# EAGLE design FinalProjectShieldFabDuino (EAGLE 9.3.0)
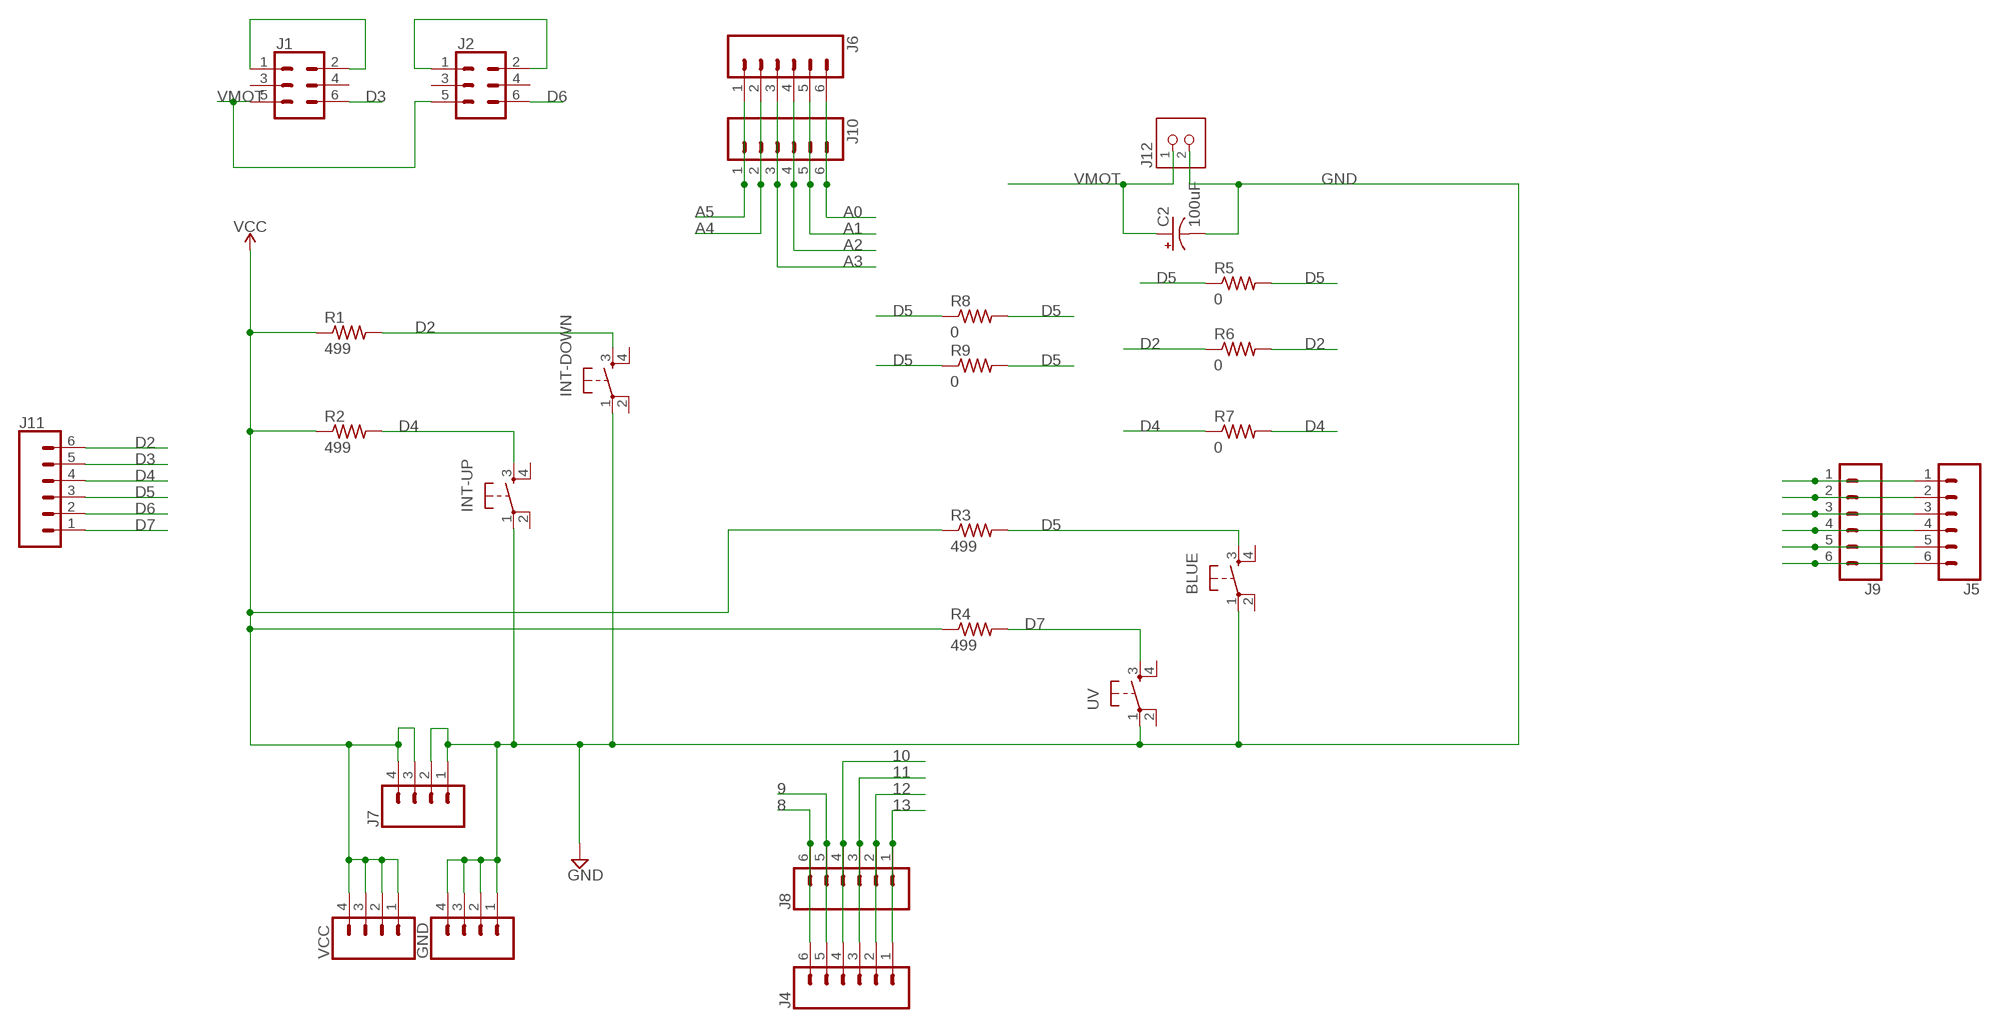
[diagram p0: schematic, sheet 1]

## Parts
BLUE  6MM_SWITCH6MM_SWITCH  [6MM_SWITCH]
C2  100uF  SPARKFUN-CAPACITORS_100UF-POLAR-RADIAL-2.5MM-25V-20%  [SPARKFUN-CAPACITORS_CPOL-RADIAL-2.5MM-6.5MM]
GND  CONN_04PTH  [1X04]
INT-DOWN  6MM_SWITCH6MM_SWITCH  [6MM_SWITCH]
INT-UP  6MM_SWITCH6MM_SWITCH  [6MM_SWITCH]
J1  CONN_03X2FEMALE_SMD  [2X3_SMD]
J2  CONN_03X2FEMALE_SMD  [2X3_SMD]
J4  CONN_06SILK_FEMALE_PTH  [1X06]
J5  CONN_06SILK_FEMALE_PTH  [1X06]
J6  CONN_06SILK_FEMALE_PTH  [1X06]
J7  SPARKFUN-CONNECTORS_CONN_04PTH  [SPARKFUN-CONNECTORS_1X04]
J8  CONN_06FEMALE_LOCK  [1X06_FEMALE_LOCK.010]
J9  CONN_06FEMALE_LOCK  [1X06_FEMALE_LOCK.010]
J10  CONN_06FEMALE_LOCK  [1X06_FEMALE_LOCK.010]
J11  CONN_06FEMALE_LOCK  [1X06_FEMALE_LOCK.010]
J12  FAB_TERM-1X02-ADAFRUIT  [FAB_3.5MMTERM]
R1  499  RES-US1206FAB  [R1206FAB]
R2  499  RES-US1206FAB  [R1206FAB]
R3  499  RES-US1206FAB  [R1206FAB]
R4  499  RES-US1206FAB  [R1206FAB]
R5  0  RES-US1206FAB  [R1206FAB]
R6  0  RES-US1206FAB  [R1206FAB]
R7  0  RES-US1206FAB  [R1206FAB]
R8  0  RES-US1206FAB  [R1206FAB]
R9  0  RES-US1206FAB  [R1206FAB]
UV  6MM_SWITCH6MM_SWITCH  [6MM_SWITCH]
VCC  CONN_04PTH  [1X04]

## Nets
8: J4.6 J8.6
9: J4.5 J8.5
10: J4.4 J8.4
11: J4.3 J8.3
12: J4.2 J8.2
13: J4.1 J8.1
A0: J6.6 J10.6
A1: J6.5 J10.5
A2: J6.4 J10.4
A3: J6.3 J10.3
A4: J6.2 J10.2
A5: J6.1 J10.1
D2: INT-DOWN.3(S) J11.6 R1.2 R6.1 R6.2
D3: J1.6 J11.5
D4: INT-UP.3(S) J11.4 R2.2 R7.1 R7.2
D5: BLUE.3(S) J11.3 R3.2 R5.1 R5.2 R8.1 R8.2 R9.1 R9.2
D6: J2.6 J11.2
D7: J11.1 R4.2 UV.3(S)
GND: BLUE.1(P) C2.2(-) GND.1 GND.2 GND.3 GND.4 INT-DOWN.1(P) INT-UP.1(P) J7.1 J7.2 J12.2 UV.1(P)
N$1: J1.1 J1.2
N$2: J2.1 J2.2
N$13: J5.1 J9.1
N$14: J5.2 J9.2
N$15: J5.3 J9.3
N$16: J5.4 J9.4
N$17: J5.5 J9.5
N$18: J5.6 J9.6
VCC: J7.3 J7.4 R1.1 R2.1 R3.1 R4.1 VCC.1 VCC.2 VCC.3 VCC.4
VMOT: C2.1(+) J1.5 J2.5 J12.1
Unconnected: BLUE.2(P1) BLUE.4(S1) INT-DOWN.2(P1) INT-DOWN.4(S1) INT-UP.2(P1) INT-UP.4(S1) J1.3 J1.4 J2.3 J2.4 UV.2(P1) UV.4(S1)

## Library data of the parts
BLUE INT-DOWN INT-UP UV = fab:6MM_SWITCH: OMRON SWITCH
C2 = GRBLShieldFabDuino:SPARKFUN-CAPACITORS_100UF-POLAR: 100µF polarized capacitors; PROD_ID: CAP-08439
GND VCC = SparkFun-Connectors:CONN_04: Multi connection point. Often used as Generic Header-pin footprint for 0.1 inch spaced/style header connections On any of the 0.1 inch spaced packages, you can populate with these: Break Away Headers - Straight (PRT-00116) Break Away Male Headers - Right Angle (PRT-00553) Female Headers (PRT-00115)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; PROD_ID: CONN-09696
J1 J2 = fab:CONN_03X2: Multi connection point. Often used as Generic Header-pin footprint for 0.1 inch spaced/style header connections You can populate with any combo of single row headers, but if you'd like an exact match, check these: Header - 2x3 (Male, 0.1") (PRT-12807) Header - 2x3 (Female, 0.1") (PRT-13010) 2x3 Pin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; PROD_ID: CONN-11290
J4-J6 = SparkFun-Connectors:CONN_06: Multi connection point. Often used as Generic Header-pin footprint for 0.1 inch spaced/style header connections On any of the 0.1 inch spaced packages, you can populate with these: Break Away Headers - Straight (PRT-00116) Break Away Male Headers - Right Angle (PRT-00553) Female Headers (PRT-00115)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; PROD_ID: CONN-08437
J7 = GRBLShieldFabDuino:SPARKFUN-CONNECTORS_CONN_04: Multi connection point. Often used as Generic Header-pin footprint for 0.1 inch spaced/style header connections On any of the 0.1 inch spaced packages, you can populate with these: Break Away Headers - Straight (PRT-00116) Break Away Male Headers - Right Angle (PRT-00553) Female Headers (PRT-00115)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; PROD_ID: CONN-09696
J8-J11 = SparkFun-Connectors:CONN_06: Multi connection point. Often used as Generic Header-pin footprint for 0.1 inch spaced/style header connections On any of the 0.1 inch spaced packages, you can populate with these: Break Away Headers - Straight (PRT-00116) Break Away Male Headers - Right Angle (PRT-00553) Female Headers (PRT-00115)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
J12 = GRBLShieldFabDuino:FAB_TERM-1X02: 3.5mm terminal block, 2 positions ED555-2DS as found in the fablab inventory.
R1-R9 = fab:RES-US: Resistor (US Symbol)

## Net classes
0 default: clearance 0.406 mm

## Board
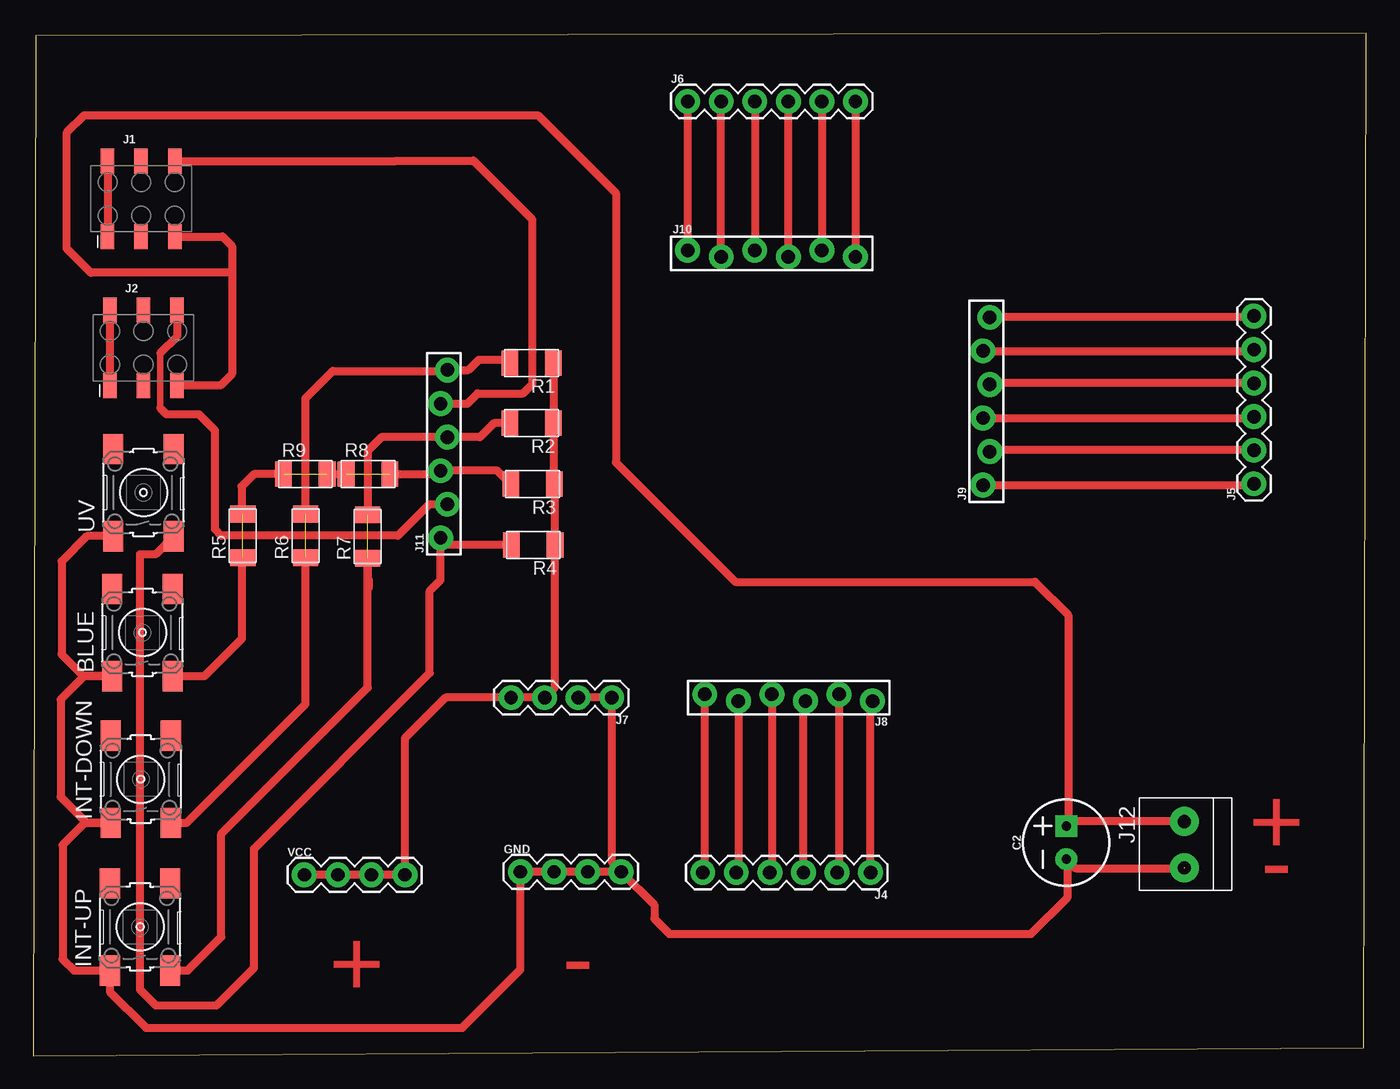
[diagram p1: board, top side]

Size 100.89 x 77.39 mm. Coordinates in mm from the lower left corner, seen from the top.
Outline: 0,0 100.69,0.61 100.89,77.39 0.2,77.19 0,0
Copper layers (1*16): Top 0.035mm / dielectric 1.5mm / Bottom 0.035mm
Design rules "default": minimum track width 6mil, minimum drill 0.35mm, track to track 6mil, track to pad 6mil, pad to pad 6mil, via to via 6mil, smd to smd 6mil, copper to edge 40mil, drill to drill 6mil, minimum pad ring 10mil, minimum via ring 8mil, stop-mask expansion 4mil, vias tented up to drill 0mil, thermal gap 10mil

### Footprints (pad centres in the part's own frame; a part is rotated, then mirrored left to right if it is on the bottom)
6MM_SWITCH = smd 2.286 x 1.524: 1 -3.302,2.286; 2 3.302,2.286; 3 -3.302,-2.286; 4 3.302,-2.286
SPARKFUN-CAPACITORS_CPOL-RADIAL-2.5MM-6.5MM = drill 0.7 pad 1.651 square: 1 1.25,0 | drill 0.7 pad 1.651: 2 -1.25,0
1X04 = drill 1.016 pad 1.88: 1 0,0; 2 2.54,0; 3 5.08,0; 4 7.62,0
2X3_SMD = smd 1.02 x 1.9: 1 -2.54,-2.85; 2 -2.54,2.85; 3 0,-2.85; 4 0,2.85; 5 2.54,-2.85; 6 2.54,2.85
1X06 = drill 1.016 pad 1.88: 1 0,0; 2 2.54,0; 3 5.08,0; 4 7.62,0; 5 10.16,0; 6 12.7,0
SPARKFUN-CONNECTORS_1X04 = drill 1.016 pad 1.88: 1 0,0; 2 2.54,0; 3 5.08,0; 4 7.62,0
1X06_FEMALE_LOCK.010 = drill 1.016 pad 1.88: 1 0,0.254; 2 2.54,-0.254; 3 5.08,0.254; 4 7.62,-0.254; 5 10.16,0.254; 6 12.7,-0.254
FAB_3.5MMTERM = drill 1 pad 2.184: 1 1.8,0; 2 -1.7,0
R1206FAB = smd 1.27 x 1.905: 1 -1.651,0; 2 1.651,0

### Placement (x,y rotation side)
BLUE  8.28,32.03 90 top
C2  78.18,16.13 90 top
GND  36.88,13.92 0 top
INT-DOWN  8.15,20.93 90 top
INT-UP  8.1,9.75 90 top
J1  8.18,64.85 0 top
J2  8.36,53.57 0 top
J4  63.37,13.87 180 top
J5  92.38,43.28 90 top
J6  49.53,72.21 0 top
J7  43.79,27.1 180 top
J8  63.53,27.1 180 top
J9  72.14,43.18 90 top
J10  49.53,60.71 0 top
J11  31.09,39.19 90 top
J12  87.12,15.93 90 top
R1  37.72,52.43 180 top
R2  37.72,47.88 180 top
R3  37.8,43.26 180 top
R4  37.85,38.66 180 top
R5  15.88,39.34 90 top
R6  20.62,39.34 90 top
R7  25.32,39.29 90 top
R8  25.35,44.02 0 top
R9  20.6,44.02 0 top
UV  8.36,42.62 90 top
VCC  20.52,13.69 0 top

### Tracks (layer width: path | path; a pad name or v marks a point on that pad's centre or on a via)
8
  Top 0.61: J4.6 50.83,14.02 J8.6
9
  Top 0.61: J8.5 53.37,14.02 J4.5
10
  Top 0.61: J8.4 55.91,14.02 J4.4
11
  Top 0.61: J4.3 58.29,26.7 J8.3
12
  Top 0.61: J8.2 60.99,14.27 61.39,13.87 61.39,13.97 61.29,13.87 J4.2
13
  Top 0.61: J4.1 63.37,26.7 J8.1
A0
  Top 0.61: J6.6 J10.6
A1
  Top 0.61: J6.5 J10.5
A2
  Top 0.61: J10.4 J6.4
A3
  Top 0.61: J6.3 J10.3
A4
  Top 0.61: J10.2 J6.2
A5
  Top 0.61: J6.1 J10.1
D2  (1 unrouted)
  Top 0.61: R1.2 35.81,52.68 33.73,52.68 32.94,51.89 J11.6 31.27,51.82 22.68,51.82 20.62,49.76 R6.2 | INT-DOWN.3 11.63,17.63 20.62,26.62 R6.1
D3
  Top 0.61: J1.6 26.59,67.7 27.38,67.7 33.28,67.7 33.32,67.74 37.79,63.27 37.79,50.83 37.08,50.11 33.63,50.11 32.87,49.35 J11.5
D4  (1 unrouted)
  Top 0.61: R2.2 34.87,47.88 33.81,46.81 J11.4 26.36,46.81 25.32,45.77 R7.2 | INT-UP.3 11.71,6.45 14.25,8.99 14.25,16.8 25.32,27.87 R7.1 25.32,35.51 25.43,35.41 25.43,36.02
D5  (3 unrouted)
  Top 0.61: R3.2 35.13,44.27 J11.3 30.58,44.02 R8.2 | BLUE.3 12.98,28.73 15.8,31.55 15.8,37.62 R5.1 | R9.1 16.71,44.02 15.77,43.08 15.77,41.1 R5.2 | R9.2 R8.1
D6
  Top 0.508: 9.62,53.16 9.62,49.02
  Top 0.61: J2.6 10.9,54.43 9.62,53.16 | 9.62,49.02 10.09,48.55 12.54,48.55 13.77,47.32 13.77,39.85 14.25,39.37 27.61,39.37 29.97,41.73 J11.2 31.32,41.71
D7
  Top 0.61: R4.2 31.37,38.66 J11.1 | 10.87,39.24 10.79,39.32 UV.3 9.27,37.95 8.08,37.95 8.08,5.03 9.3,3.81 13.89,3.81 16.73,6.64 16.73,15.66 30.02,28.96 30.02,35.18 30.84,35.99 J11.1 | 30.78,39.24 J11.1
GND  (1 unrouted)
  Top 0.61: C2.2 78.29,14.77 | 78.29,14.77 78.86,14.2 87.15,14.2 87.2,14.15 | GND.4 GND.3 GND.2 GND.1 36.88,6.53 32.47,2.12 8.55,2.12 5.82,4.85 INT-UP.1 3.1,6.45 2.23,7.31 2.23,15.95 3.91,17.63 INT-DOWN.1 4.06,17.63 2.08,19.61 2.08,26.95 3.86,28.73 BLUE.1 3.81,28.73 2.16,30.38 2.16,37.41 4.06,39.32 UV.1 | GND.4 44.5,13.97 43.79,14.68 J7.1 J7.2 | GND.4 47.02,11.4 47.02,10.36 48.16,9.22 75.51,9.22 78.29,12 78.29,14.77
N$1
  Top 0.61: J1.2 J1.1
N$2
  Top 0.61: J2.2 J2.1
N$13
  Top 0.61: J9.1 92.28,43.18 J5.1
N$14
  Top 0.61: J5.2 72.49,45.82 J9.2
N$15
  Top 0.61: J9.3 92.28,48.26 J5.3
N$16
  Top 0.61: J5.4 72.49,50.9 J9.4
N$17
  Top 0.61: J9.5 92.91,53.34 92.94,53.37 92.86,53.44 J5.5
N$18
  Top 0.61: J5.6 92.28,55.88 J9.6
VCC
  Top 0.61: VCC.1 VCC.2 VCC.3 VCC.4 28.12,13.72 28.12,24 31.22,27.1 J7.4 J7.3 39.5,27.89 R4.1 39.45,38.71 R3.1 39.37,43.33 R2.1 R1.1
VMOT
  Top 0.61: 78.33,17.53 78.53,17.73 J12.1 87.15,17.75 | 78.33,17.53 C2.1 | J1.5 14.33,62 15.06,61.26 15.06,59.26 | 15.06,59.26 15.06,51.59 14.19,50.72 J2.5 | 15.06,59.26 4.37,59.26 2.55,61.08 2.57,69.88 3.86,71.17 38.2,71.17 44.09,65.28 44.09,44.91 53.14,35.86 75.82,35.86 78.33,33.35 78.33,17.53

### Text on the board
Top: + | - | - | +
